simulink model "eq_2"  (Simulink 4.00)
settings: Solver=ode45  StartTime=0.0  StopTime=10.0  RelTol=1e-3
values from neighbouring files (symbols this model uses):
  csi = 0.09    [RotFilo.m]
  g = 9.81    [RotFilo.m]
  L = 0.3    [RotFilo.m]
  mu = E*A/2/T0    (= 0.00237504404611)    [RotFilo.m]
  r = w/w0    [RotFilo.m]
  w = 2*pi*n/60    (= 314.159265359)    [RotFilo.m]

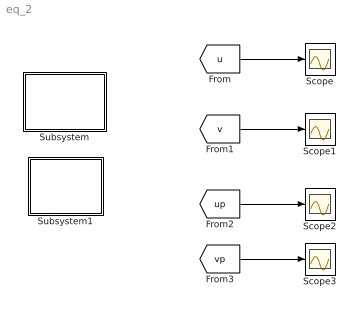
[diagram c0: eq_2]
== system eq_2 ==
  Scope{,1..3} (4 alike) : Scope
  Subsystem : Subsystem
  Subsystem1 : Subsystem
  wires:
  [u] -> Scope/1
  [v] -> Scope1/1
  [up] -> Scope2/1
  [vp] -> Scope3/1

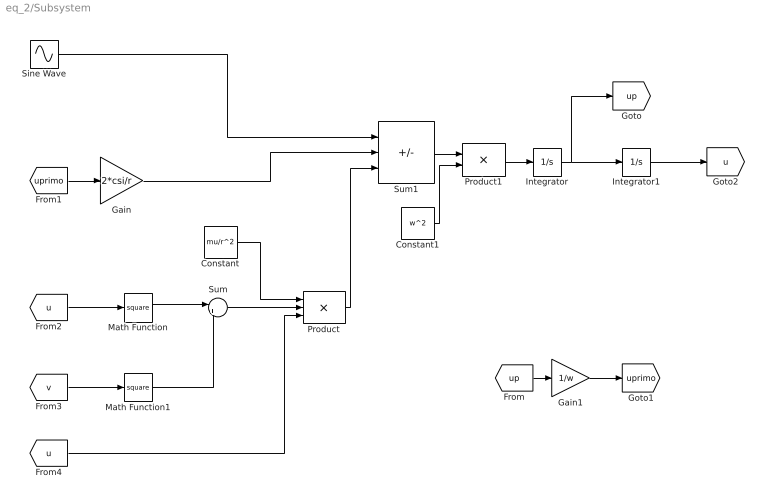
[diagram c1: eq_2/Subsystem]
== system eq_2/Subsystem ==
  Constant : Constant  Value=mu/r^2
  Constant1 : Constant  Value=w^2
  Gain : Gain  Gain=2*csi/r  Multiplication=Element-wise(K.*u)  SaturateOnIntegerOverflow=on
  Gain1 : Gain  Gain=1/w  Multiplication=Element-wise(K.*u)  SaturateOnIntegerOverflow=on
  Integrator : Integrator  ExternalReset=none  InitialConditionSource=internal  InitialCondition=0  LimitOutput=off  UpperSaturationLimit=inf  LowerSaturationLimit=-inf  ShowSaturationPort=off  ShowStatePort=off  AbsoluteTolerance=auto
  Integrator1 : Integrator  ExternalReset=none  InitialConditionSource=internal  InitialCondition=0  LimitOutput=off  UpperSaturationLimit=inf  LowerSaturationLimit=-inf  ShowSaturationPort=off  ShowStatePort=off  AbsoluteTolerance=auto
  Math Function : Math  Operator=square  OutputSignalType=auto
  Math Function1 : Math  Operator=square  OutputSignalType=auto
  Product : Product  Inputs=3  Multiplication=Element-wise(.*)  SaturateOnIntegerOverflow=on
  Product1 : Product  Inputs=2  Multiplication=Element-wise(.*)  SaturateOnIntegerOverflow=on
  Sine Wave : Sin  SineType=Time-based  Amplitude=e/L  Bias=0  Frequency=w  Phase=pi/2  Samples=10  SampleTime=0
  Sum : Sum  Inputs=|++  SaturateOnIntegerOverflow=on
  Sum1 : Sum  Inputs=+--  SaturateOnIntegerOverflow=on
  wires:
  Integrator/1 -> Integrator1/1, [up]
  [up] -> Gain1/1
  Gain1/1 -> [uprimo]
  [uprimo] -> Gain/1
  Integrator1/1 -> [u]
  [u] -> Math Function/1
  [v] -> Math Function1/1
  Math Function/1 -> Sum/1
  Math Function1/1 -> Sum/2
  Sum/1 -> Product/2
  [u] -> Product/3
  Constant/1 -> Product/1
  Sine Wave/1 -> Sum1/1
  Gain/1 -> Sum1/2
  Product/1 -> Sum1/3
  Product1/1 -> Integrator/1
  Sum1/1 -> Product1/1
  Constant1/1 -> Product1/2

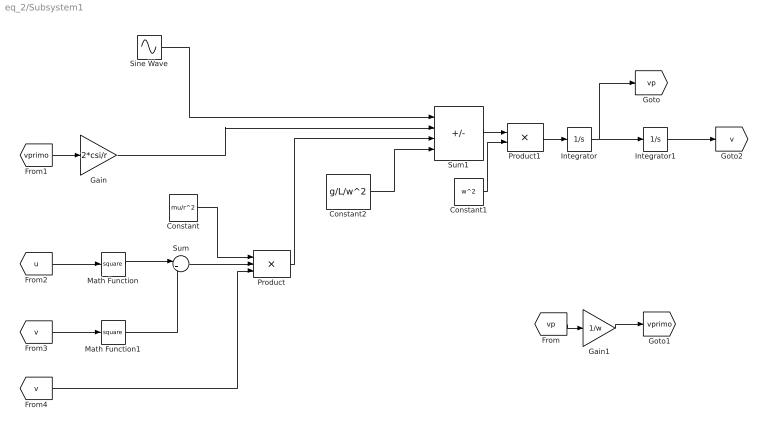
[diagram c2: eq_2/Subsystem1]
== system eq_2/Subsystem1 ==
  Constant : Constant  Value=mu/r^2
  Constant1 : Constant  Value=w^2
  Constant2 : Constant  Value=g/L/w^2
  Gain : Gain  Gain=2*csi/r  Multiplication=Element-wise(K.*u)  SaturateOnIntegerOverflow=on
  Gain1 : Gain  Gain=1/w  Multiplication=Element-wise(K.*u)  SaturateOnIntegerOverflow=on
  Integrator : Integrator  ExternalReset=none  InitialConditionSource=internal  InitialCondition=0  LimitOutput=off  UpperSaturationLimit=inf  LowerSaturationLimit=-inf  ShowSaturationPort=off  ShowStatePort=off  AbsoluteTolerance=auto
  Integrator1 : Integrator  ExternalReset=none  InitialConditionSource=internal  InitialCondition=0  LimitOutput=off  UpperSaturationLimit=inf  LowerSaturationLimit=-inf  ShowSaturationPort=off  ShowStatePort=off  AbsoluteTolerance=auto
  Math Function : Math  Operator=square  OutputSignalType=auto
  Math Function1 : Math  Operator=square  OutputSignalType=auto
  Product : Product  Inputs=3  Multiplication=Element-wise(.*)  SaturateOnIntegerOverflow=on
  Product1 : Product  Inputs=2  Multiplication=Element-wise(.*)  SaturateOnIntegerOverflow=on
  Sine Wave : Sin  SineType=Time-based  Amplitude=e/L  Bias=0  Frequency=w  Phase=0  Samples=10  SampleTime=0
  Sum : Sum  Inputs=|++  SaturateOnIntegerOverflow=on
  Sum1 : Sum  Inputs=+---  SaturateOnIntegerOverflow=on
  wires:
  Integrator/1 -> Integrator1/1, [vp]
  [vp] -> Gain1/1
  Gain1/1 -> [vprimo]
  [vprimo] -> Gain/1
  Integrator1/1 -> [v]
  [u] -> Math Function/1
  [v] -> Math Function1/1
  Math Function/1 -> Sum/1
  Math Function1/1 -> Sum/2
  Sum/1 -> Product/2
  [v] -> Product/3
  Constant/1 -> Product/1
  Sine Wave/1 -> Sum1/1
  Gain/1 -> Sum1/2
  Product/1 -> Sum1/3
  Product1/1 -> Integrator/1
  Sum1/1 -> Product1/1
  Constant1/1 -> Product1/2
  Constant2/1 -> Sum1/4
